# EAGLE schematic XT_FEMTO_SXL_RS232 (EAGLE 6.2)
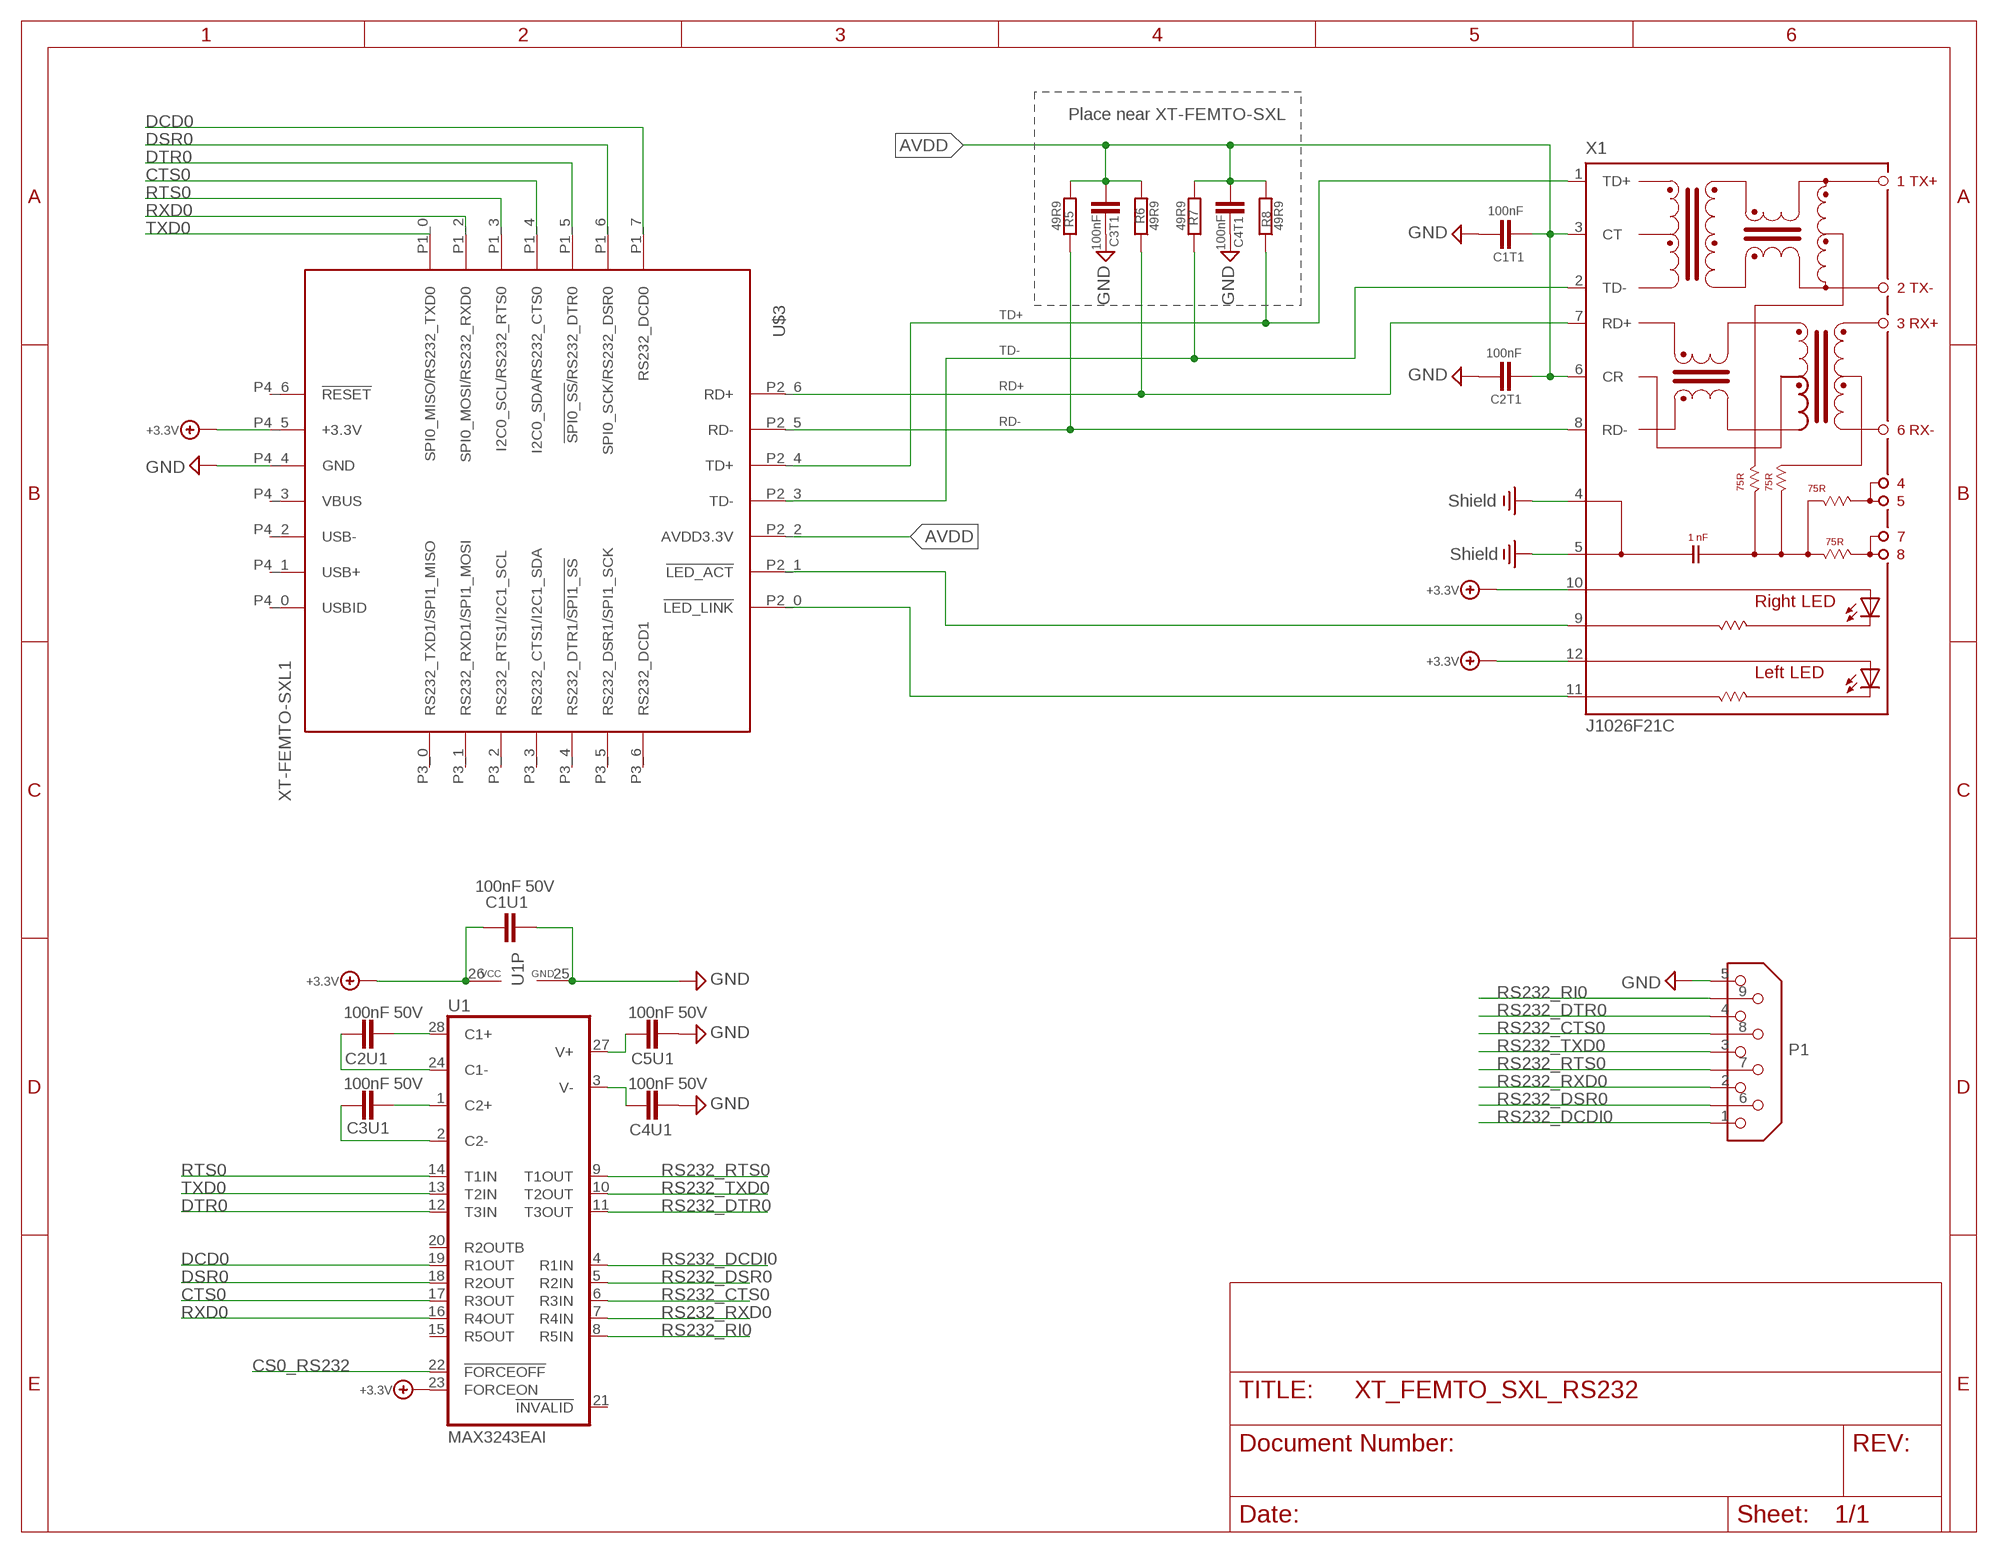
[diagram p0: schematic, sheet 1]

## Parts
C1T1  100nF  CHIP-C-VTS0402  [R0402_VTS]
C1U1  100nF 50V  CHIP-C-0603  [SMD-0603]
C2T1  100nF  CHIP-C-VTS0402  [R0402_VTS]
C2U1  100nF 50V  CHIP-C-0603  [SMD-0603]
C3T1  100nF  CHIP-C-VTS0402  [R0402_VTS]
C3U1  100nF 50V  CHIP-C-0603  [SMD-0603]
C4T1  100nF  CHIP-C-VTS0402  [R0402_VTS]
C4U1  100nF 50V  CHIP-C-0603  [SMD-0603]
C5U1  100nF 50V  CHIP-C-0603  [SMD-0603]
P1  DB9  [MSUB9-5]
R5  49R9  R-EU_R0603  [R0603]
R6  49R9  R-EU_R0603  [R0603]
R7  49R9  R-EU_R0603  [R0603]
R8  49R9  R-EU_R0603  [R0603]
U1  MAX3243EAI  [SSOP28]
U$3  XT-FEMTO-SXL1  [XT-FEMTO-SXL-PIN]
X1  J1026F21C  [J1]

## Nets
+3.3V: C1U1.1 U1.23(FORCEON) U1.26(VCC) U$3.P4_5(+3.3V) X1.10(A-R) X1.12(A-L)
AVDD: C1T1.1 C2T1.2 C3T1.1 C4T1.2 R5.2 R6.2 R7.2 R8.2 U$3.P2_2(AVDD3.3V) X1.3(CT) X1.6(CR)
CS0_RS232: U1.22(!FORCEOFF)
CTS0: U1.17(R3OUT) U$3.P1_4(I2C0_SDA/RS232_CTS0)
DCD0: U1.19(R1OUT) U$3.P1_7(RS232_DCD0)
DSR0: U1.18(R2OUT) U$3.P1_6(SPI0_SCK/RS232_DSR0)
DTR0: U1.12(T3IN) U$3.P1_5(!SPI0_SS!/RS232_DTR0)
GND: C1T1.2 C1U1.2 C2T1.1 C3T1.2 C4T1.1 C4U1.2 C5U1.2 P1.5 U1.25(GND) U$3.P4_4(GND)
N$3: U$3.P2_1(!LED_ACT) X1.9(C-R)
N$5: U$3.P2_0(!LED_LINK) X1.11(C-L)
N$22: C4U1.1 U1.3(V-)
N$23: C5U1.1 U1.27(V+)
N$24: C3U1.2 U1.1(C2+)
N$26: C2U1.2 U1.28(C1+)
N$27: C3U1.1 U1.2(C2-)
N$28: C2U1.1 U1.24(C1-)
PE: X1.4 X1.5 ; supply symbol labelled Shield
RD+: R6.1 U$3.P2_6(RD+) X1.7(RD+)
RD-: R5.1 U$3.P2_5(RD-) X1.8(RD-)
RS232_CTS0: P1.8 U1.6(R3IN)
RS232_DCDI0: P1.1 U1.4(R1IN)
RS232_DSR0: P1.6 U1.5(R2IN)
RS232_DTR0: P1.4 U1.11(T3OUT)
RS232_RI0: P1.9 U1.8(R5IN)
RS232_RTS0: P1.7 U1.9(T1OUT)
RS232_RXD0: P1.2 U1.7(R4IN)
RS232_TXD0: P1.3 U1.10(T2OUT)
RTS0: U1.14(T1IN) U$3.P1_3(I2C0_SCL/RS232_RTS0)
RXD0: U1.16(R4OUT) U$3.P1_2(SPI0_MOSI/RS232_RXD0)
TD+: R8.1 U$3.P2_4(TD+) X1.1(TD+)
TD-: R7.1 U$3.P2_3(TD-) X1.2(TD-)
TXD0: U1.13(T2IN) U$3.P1_0(SPI0_MISO/RS232_TXD0)
Unconnected: U1.15(R5OUT) U1.20(R2OUTB) U1.21(!INVALID) U$3.P3_0(RS232_TXD1/SPI1_MISO) U$3.P3_1(RS232_RXD1/SPI1_MOSI) U$3.P3_2(RS232_RTS1/I2C1_SCL) U$3.P3_3(RS232_CTS1/I2C1_SDA) U$3.P3_4(RS232_DTR1/!SPI1_SS!) U$3.P3_5(RS232_DSR1/SPI1_SCK) U$3.P3_6(RS232_DCD1) U$3.P4_0(USBID) U$3.P4_1(USB+) U$3.P4_2(USB-) U$3.P4_3(VBUS) U$3.P4_6(!RESET)

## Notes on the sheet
- Place near XT-FEMTO-SXL

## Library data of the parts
C1T1 C1U1 C2T1 C2U1 C3T1 C3U1 C4T1 C4U1 C5U1 = mea-lib:CHIP-C-?: Chip capacitance
P1 = XTMACRO:DB9
R5-R8 = rcl:R-EU_: RESISTOR, European symbol
U1 = maxim:MAX3243*: RS-232 Transceivers with AutoShutdown 1µA Supply-Current, True +3V to +5.5V http://dbserv.maxim-ic.com/
U$3 = ak-devices:XT-FEMTO-SXL: AK-NORD XT-FEMTO-SXL
X1 = con-pulse:J1026F: PULSEJACK (TM) 1x1 Tab-UP RJ45 10/100 Base-TX RJ45 1x1 Tab-UP with LEDs 8-pin (J1 series) and 6-pin (JP series) integrated magnetics connector, designed to support applications, such as ADSL modems, LAN-on-Motherboard, and Hub and Switches. Source: www.pulseeng.com .. PulseJack-J402.pdf; OC_FARNELL: unknown; OC_NEWARK: unknown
